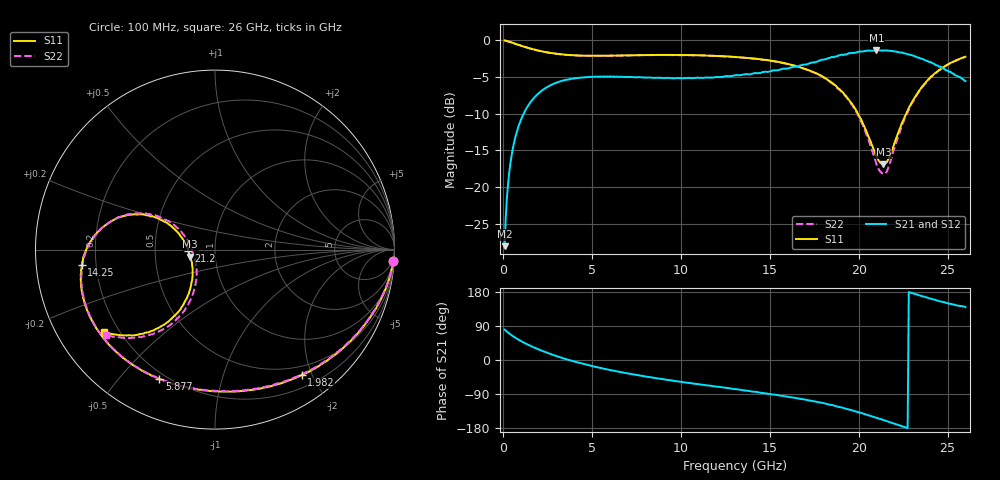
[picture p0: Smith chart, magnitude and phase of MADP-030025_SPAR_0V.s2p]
!Mean
# HZ S DB R 50
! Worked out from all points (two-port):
!   400 points, 100 MHz to 26 GHz, reference 50 ohm
!   highest |S21| = -1.37 dB at 21 GHz (marker M1); lowest = -28.0 dB at 100 MHz (marker M2)
!   |S21| within 3 dB of the highest: 14.57 GHz to 25.2 GHz (10.62 GHz wide, 53.4 % of centre)
!   lowest |S11| = -16.9 dB at 21.39 GHz (marker M3), VSWR 1.33, Z = 37.8 - j3.08 ohm
!   |S11| at or under -10 dB: 19.96 GHz to 22.67 GHz (2.71 GHz wide, 12.7 % of centre)
!   |S22| runs from -18.2 to 0.0 dB; largest |S21 - S12| = 0.0074
!   S11 on the Smith chart (normalised r, x): 100 MHz: 2, -30; 1.982 GHz: 0.37, -1.85; 5.877 GHz: 0.17, -0.64; 14.25 GHz: 0.14, -0.06; 21.2 GHz: 0.74, -0.01; 26 GHz: 0.14, -0.32
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1e8  -0.04 -3.8  -28.03 80.2  -28.03 79.8  -0.04 -3.7
1.6491e8  -0.07 -6.1  -24.08 77.2  -24.08 77.2  -0.07 -6.0
2.9474e8  -0.16 -10.5  -19.56 72.3  -19.54 72.2  -0.17 -10.3
6.193e8  -0.42 -20.8  -14.08 61.2  -14.08 61.1  -0.42 -20.3
1.1386e9  -0.85 -35.3  -10.16 46.8  -10.16 46.8  -0.86 -34.5
1.9825e9  -1.41 -55.3  -7.29 28.4  -7.28 28.5  -1.41 -53.9
3.086e9  -1.87 -76.5  -5.72 9.2  -5.72 9.2  -1.88 -74.8
4.4491e9  -2.10 -96.7  -5.07 -9.4  -5.07 -9.4  -2.11 -94.9
5.8772e9  -2.11 -113.3  -4.94 -25.0  -4.95 -25.0  -2.13 -111.6
8.7982e9  -2.00 -138.7  -5.10 -49.1  -5.11 -49.2  -2.03 -137.3
1.3082e10  -2.29 -166.5  -4.78 -76.9  -4.80 -77.0  -2.30 -165.8
1.4251e10  -2.53 -173.5  -4.47 -84.2  -4.53 -84.3  -2.55 -173.0
1.7367e10  -4.25 166.2  -3.05 -107.7  -3.06 -107.6  -4.29 165.9
1.9639e10  -8.71 151.2  -1.73 -132.8  -1.78 -133.0  -8.85 149.4
2.1002e10  -15.86 171.6  -1.37 -152.7  -1.36 -152.6  -16.89 168.3
2.1196e10  -16.59 -176.8  -1.39 -155.4  -1.39 -155.4  -17.85 -178.5
2.1391e10  -16.88 -163.8  -1.38 -158.5  -1.38 -158.5  -18.21 -163.3
2.1716e10  -15.96 -142.1  -1.43 -163.6  -1.44 -163.5  -17.05 -137.6
2.2625e10  -10.23 -120.1  -1.80 -177.7  -1.81 -177.5  -10.47 -116.0
2.3533e10  -6.44 -122.8  -2.52 168.9  -2.49 169.0  -6.52 -119.9
2.4572e10  -4.00 -131.8  -3.60 154.4  -3.58 154.8  -4.05 -129.6
2.6e10  -2.25 -143.6  -5.57 139.5  -5.47 139.6  -2.27 -142.0
